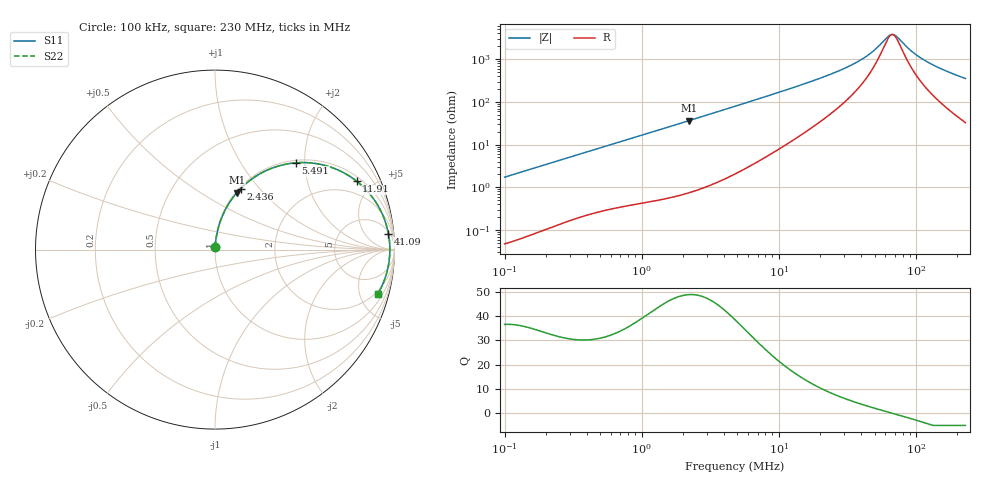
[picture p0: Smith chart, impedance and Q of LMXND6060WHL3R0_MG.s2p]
! LMXND6060WHL3R0_MG  S-PARAMETER MODEL  ( General Type )
! Model Generated by TAIYO YUDEN Corporation (https://www.yuden.co.jp/en/)
! Version 1.0
! TAIYO YUDEN Control No. 191025NI43SB-FBB
! Copyright(c) 2019 TAIYO YUDEN CO.,LTD. All Rights Reserved.
! Product Description (link to TY-COMPAS)
! https://ds.yuden.co.jp/TYCOMPAS/or/detail?pn=LMXND6060WHL3R0NMG&u=M
! Products Name : Inductors
! Characteristics :
!  Inductance : 3.0 uH , SRF(min) : 55 MHz , DC Resistance(max) : 0.0299 Ohm
!  Rated Current : Saturation :3600 mA , Temp Rise : 3400 mA (40 degC)
!  Case Size : 6.0 x 6.0 / 0.236 x 0.236 [mm/inch] , Thickness : 2.8 / 0.11 [mm/inch]
!  (Conditions: Temperature = 25 degC , DC Bias Current/Voltage = 0A / 0V)
! External Node Assignments :
!  1  o---GGG---o  2
! GND o---------o GND
! Frequency Range : 0.1MHz  -  229.966873MHz  [ 402 STEP ]
# MHz S RI R 50
! Freq[MHz].  S11 Real  S11 Imag  S21 Real  S21 Imag  S12 Real  S12 Imag  S22 Real  S22 Imag
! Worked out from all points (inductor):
!   401 points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, 100 kHz to 230 MHz, reference 50 ohm
!   read as one part in series: L = 2.74 uH near 103.9 kHz
!   highest Q = 48.8 at 2.211 MHz (marker M1), where L = 2.61 uH
!   self-resonance near 67.39 MHz
!   S11 on the Smith chart (normalised r, x): 100 kHz: 1.00, +0.03; 2.436 MHz: 1.02, +0.80; 5.491 MHz: 1.05, +1.81; 11.91 MHz: 1.22, +4.01; 41.09 MHz: 7, +20; 230 MHz: 1.65, -7.01
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0.1  0.00077 0.0173  0.9992 -0.0173  0.9992 -0.0173  0.00077 0.0173
0.365661  0.00582 0.0613  0.9942 -0.0613  0.9942 -0.0613  0.00582 0.0613
0.733886  0.018 0.1192  0.982 -0.1192  0.982 -0.1192  0.018 0.1192
1.337081  0.0505 0.2079  0.9495 -0.2079  0.9495 -0.2079  0.0505 0.2079
2.211394  0.1215 0.3166  0.8785 -0.3166  0.8785 -0.3166  0.1215 0.3166
2.436054  0.143 0.34  0.857 -0.34  0.857 -0.34  0.143 0.34
3.384992  0.241 0.4169  0.759 -0.4169  0.759 -0.4169  0.241 0.4169
4.889189  0.3959 0.4761  0.6041 -0.4761  0.6041 -0.4761  0.3959 0.4761
5.491131  0.4517 0.4837  0.5483 -0.4837  0.5483 -0.4837  0.4517 0.4837
7.779232  0.6205 0.467  0.3795 -0.467  0.3795 -0.467  0.6205 0.467
11.90771  0.7889 0.3815  0.2111 -0.3815  0.2111 -0.3815  0.7889 0.3815
17.53523  0.8854 0.2799  0.1146 -0.2799  0.1146 -0.2799  0.8854 0.2799
28.44564  0.9462 0.1626  0.0538 -0.1626  0.0538 -0.1626  0.9462 0.1626
41.08608  0.9663 0.0879  0.0337 -0.0879  0.0337 -0.0879  0.9663 0.0879
49.85818  0.9715 0.0525  0.0285 -0.0525  0.0285 -0.0525  0.9715 0.0525
64.11956  0.9743 0.00856  0.0257 -0.00856  0.0257 -0.00856  0.9743 0.00856
67.95212  0.9743 -0.00143  0.0257 0.00143  0.0257 0.00143  0.9743 -0.00143
72.01376  0.9742 -0.0114  0.0258 0.0114  0.0258 0.0114  0.9742 -0.0114
94.42213  0.9708 -0.0589  0.0292 0.0589  0.0292 0.0589  0.9708 -0.0589
121.4305  0.9627 -0.106  0.0373 0.106  0.0373 0.106  0.9627 -0.106
165.4987  0.9435 -0.1706  0.0565 0.1706  0.0565 0.1706  0.9435 -0.1706
229.9669  0.9056 -0.2494  0.0944 0.2494  0.0944 0.2494  0.9056 -0.2494
